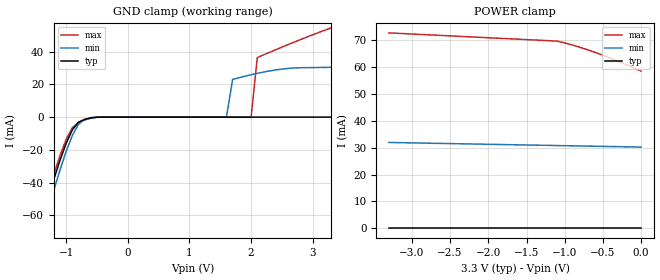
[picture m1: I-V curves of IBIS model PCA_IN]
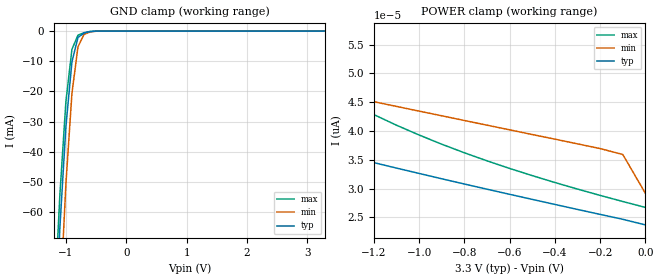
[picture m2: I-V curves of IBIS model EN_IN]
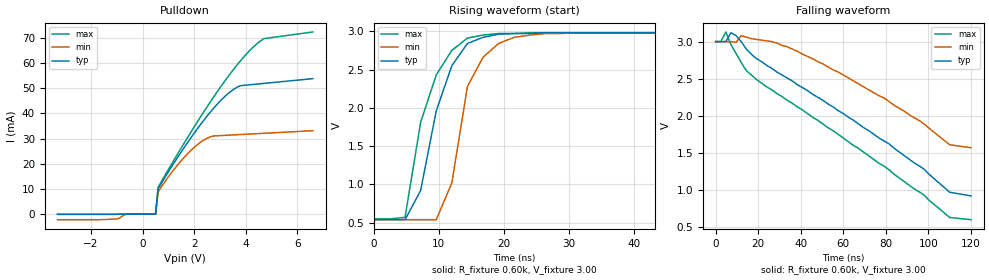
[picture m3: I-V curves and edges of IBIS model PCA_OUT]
| Philips Semiconductors Inc.
| Specialty Logic Group
| IBIS model of PCA9518
| Expandable 5-channel I2C Hub
[IBIS ver]   3.2
[File name]   pca9518.ibs
[File Rev]   1.0
[Date]   July 16, 2002
[Source]   Philips Semiconductors, Albuquerque
[Notes]   Generated by GMJ
PCA9518 IBIS MODEL
Because the PCA9518 is a repeater, not a buffer, this IBIS model does not model
the functionality of part correctly.  It only models unidirectional output
characteristics of the part. This is due to the fact that the input voltage
characteristics are affected by the voltage on the output side.
And as seen in the graph is a time dependent behavior.  This is illustrated
in the image Difference.png
[Disclaimer]
   (C) Copyright 2002 Philips Semiconductors
   All rights reserved
   Philips Semiconductors warrants and represents that the IBIS model
   identified herein is owned by Philips Semiconductors (PHILIPS). The
   model provided is not warranted as fully representing all of the
   operating characteristics and specifications of the semiconductor
   products to which the model relates.  Moreover, unless there is a
   signed, written agreement to the contrary, this IBIS model is
   furnished on an "as is" basis without support or warranty of any
   kind, either expressed or implied, regarding the use thereof, and
   PHILIPS specifically disclaims all implied warranties of
   merchantability and fitness of the model for any purpose.
   PHILIPS does not assume any liability arising out of the application
   or use of this IBIS model including infringement of patents and
   copyrights, nor does PHILIPS convey any license under its patents and
   copyrights or the rights of others.
   PHILIPS provides IBIS models as a service to our customers. You and
   your company shall not distribute, convey, sell, or give these models
   to anyone else without receiving prior written permission from
   PHILIPS.
   PHILIPS reserves the right to make changes without notice to these
   IBIS models to improve reliability, function, or design.
   Please be aware that your receipt and subsequent use of the IBIS
   information provided shall serve as acceptance of the terms and
   conditions of this agreement.  If you do not accept these terms,
   you should return or destroy the IBIS models and any other
   accompanying information immediately.
|   Component PCA9518
[Component]   PCA9518D
[Manufacturer]   Philips Semiconductors
[Package]
|[Package]   SO20
|   typ   min   max
R_pkg   5.95E-02   5.36E-02   6.59E-02
L_pkg   4.21E-09   3.07E-09   5.91E-09
C_pkg   0.910E-12  0.758E-12  1.110E-12
| Note:  All clock & data paths bidirectional.  IN/OUT choices arbitrary.
[Pin]  signal_name   model_name   R_pin   L_pin   C_pin
1   EXPSCL1   PCA_IN   5.75E-02  5.91E-09  1.050E-12
2   EXPSCL2   PCA_OUT   6.25E-02  4.85E-09  1.040E-12
3   SCL0   PCA_IN   6.59E-02  3.92E-09  0.861E-12
4   SDA0   PCA_IN   5.79E-02  3.32E-09  0.803E-12
5   SCL1   PCA_OUT   5.36E-02  3.07E-09  0.758E-12
6   SDA1   PCA_OUT   5.36E-02  3.07E-09  0.758E-12
7   EN1   EN_IN   5.79E-02  3.32E-09  0.803E-12
8   SCL2   POWER   6.59E-02  3.92E-09  0.861E-12
9   SDA2   PCA_OUT   6.25E-02  4.85E-09  1.040E-12
10   GND   PCA_OUT   5.75E-02  5.91E-09  1.110E-12
11   EN2   EN_IN   5.75E-02  5.91E-09  1.110E-12
12   SCL3   PCA_OUT   6.25E-02  4.85E-09  1.040E-12
13   SDA3   PCA_OUT   6.59E-02  3.92E-09  0.861E-12
14   EN3   EN_IN   5.79E-02  3.32E-09  0.803E-12
15   SCL4   PCA_OUT   5.36E-02  3.07E-09  0.758E-12
16   SDA4   PCA_OUT   5.36E-02  3.07E-09  0.758E-12
17   EN4   EN_IN   5.79E-02  3.32E-09  0.803E-12
18   EXPSDA1   PCA_IN   6.59E-02  3.92E-09  0.861E-12
19   EXPSDA2   PCA_OUT   6.25E-02  4.85E-09  1.040E-12
20   VCC   POWER   5.75E-02  5.91E-09  1.110E-12
[Component]   PCA9518PW
[Manufacturer]   Philips Semiconductors
[Package]
|[Package]   TSSOP20
|   typ   min   max
R_pkg   7.24E-02   6.63E-02   8.34E-02
L_pkg   2.47E-09   2.09E-09   3.18E-09
C_pkg   0.341E-12  0.282E-12  0.420E-12
| Note:  All clock & data paths bidirectional.  IN/OUT choices arbitrary.
[Pin]  signal_name   model_name   R_pin   L_pin   C_pin
1   EXPSCL1   PCA_IN   6.63E-02  3.18E-09  0.408E-12
2   EXPSCL2   PCA_OUT   6.67E-02  2.55E-09  0.398E-12
3   SCL0   PCA_IN   8.34E-02  2.35E-09  0.317E-12
4   SDA0   PCA_IN   7.44E-02  2.16E-09  0.293E-12
5   SCL1   PCA_OUT   7.10E-02  2.09E-09  0.282E-12
6   SDA1   PCA_OUT   7.10E-02  2.09E-09  0.282E-12
7   EN1   EN_IN   7.44E-02  2.16E-09  0.293E-12
8   SCL2   POWER   8.34E-02  2.35E-09  0.317E-12
9   SDA2   PCA_OUT   6.67E-02  2.55E-09  0.397E-12
10   GND   PCA_OUT   6.63E-02  3.18E-09  0.420E-12
11   EN2   EN_IN   6.63E-02  3.17E-09  0.420E-12
12   SCL3   PCA_OUT   6.67E-02  2.55E-09  0.397E-12
13   SDA3   PCA_OUT   8.34E-02  2.35E-09  0.317E-12
14   EN3   EN_IN   7.44E-02  2.16E-09  0.293E-12
15   SCL4   PCA_OUT   7.10E-02  2.09E-09  0.282E-12
16   SDA4   PCA_OUT   7.10E-02  2.09E-09  0.282E-12
17   EN4   EN_IN   7.44E-02  2.16E-09  0.293E-12
18   EXPSDA1   PCA_IN   8.34E-02  2.35E-09  0.317E-12
19   EXPSDA2   PCA_OUT   6.67E-02  2.55E-09  0.398E-12
20   VCC   POWER   6.63E-02  3.17E-09  0.420E-12
| Models and submodels in the file (3): PCA_IN (Input), EN_IN (Input), PCA_OUT (Open_drain)
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|   Model PCA_IN
[Model]   PCA_IN
Model_type   Input
Vinl =   0.50V
Vinh =   2.50V
C_comp   5.00pF   5.00pF   5.00pF
[Temperature Range]   27.00   70.00   0.000
[Voltage Range]   3.30V   3.00V   3.60V
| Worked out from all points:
|   GND clamp passes 1 mA (typ) near -0.66 V on its own axis
[GND_clamp]
| voltage   I(typ)   I(min)   I(max)
-3.3V     -340mA     -350mA     -330mA
-1.5V     -76.49mA   -84.37mA   -73.19mA
-1.4V     -63.24mA   -70.75mA   -59.96mA
-1V       -15.96mA   -20.9mA    -13.54mA
-900mV    -7.75mA    -11.17mA   -6.43mA
-800mV    -3.12mA    -4.33mA    -3.2mA
-700mV    -1.41mA    -1.29mA    -1.74mA
1.6V      29.23pA    32.44pA    29.06pA
1.7V      31.36pA    22.97mA    31.34pA
2V        37.97pA    25.86mA    38.69pA
2.1V      40.25pA    26.71mA    36.33mA
3.3V      73.63pA    30.39mA    54.51mA
[POWER_clamp]
| voltage   I(typ)   I(min)   I(max)
-3.3V     560pA      31.96mA    72.81mA
-1.1V     130pA      30.8mA     69.76mA
-1V       120pA      30.75mA    69.07mA
-900mV    110pA      30.7mA     68.29mA
-700mV    100pA      30.59mA    66.51mA
-600mV    98.17pA    30.54mA    65.52mA
-500mV    93.48pA    30.49mA    64.47mA
-300mV    84.89pA    30.39mA    62.22mA
0V        73.63pA    30.23mA    58.52mA
|   Model EN_IN
[Model]   EN_IN
Model_type   Input
Enable   Active-High
Vinl =   0.50V
Vinh =   2.50V
C_comp   5.00pF   5.00pF   5.00pF
[Temperature Range]   27.00   70.00   0.000
[Voltage Range]   3.30V   3.00V   3.60V
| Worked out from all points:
|   GND clamp passes 1 mA (typ) near -0.72 V on its own axis
[GND_clamp]
| voltage   I(typ)   I(min)   I(max)
-3.3V     -1.4A      -1.5A      -1.38A
-1.2V     -110mA     -140mA     -94.8mA
-1.1V     -65.23mA   -91.55mA   -54.4mA
-1V       -31.67mA   -50.72mA   -23.4mA
-900mV    -10.21mA   -20.66mA   -6.06mA
-800mV    -2.12mA    -5.24mA    -1.35mA
-700mV    -650uA     -1.09mA    -540uA
-600mV    -170uA     -300uA     -120uA
-500mV    -19.26uA   -44.66uA   -17.4uA
3.3V      23.67pA    37.76pA    -3.93nA
[POWER_clamp]
| voltage   I(typ)   I(min)   I(max)
-3.3V     62.39pA    62.57pA    200pA
-3V       56.74pA    60.02pA    150pA
-2.6V     50.46pA    56.65pA    100pA
-2.2V     45.18pA    53.32pA    75.29pA
-1.8V     40.59pA    50.01pA    58.19pA
-1.7V     39.52pA    49.18pA    54.97pA
-1.5V     37.45pA    47.54pA    49.44pA
-1.3V     35.47pA    45.91pA    44.86pA
-1V       32.62pA    43.45pA    39.3pA
-600mV    28.99pA    40.2pA     33.49pA
-100mV    24.65pA    35.91pA    27.74pA
0V        23.67pA    29.15pA    26.71pA
|   Model PCA_OUT
[Model]   PCA_OUT
Model_type   Open_drain
Polarity   Non-Inverting
C_comp   5.00pF   5.00pF   5.00pF
[Temperature Range]   27.00   70.00   0.000
[Voltage Range]   3.30V   3.00V   3.60V
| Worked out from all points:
|   rising waveform, R_fixture 0.60k, V_fixture 3.00: 20-80 % time 4.34ns typ, 3.77ns min, 4.43ns max; typ from 0.54 V to 2.99 V
|   falling waveform, R_fixture 0.60k, V_fixture 3.00: 20-80 % time 65.9ns typ, 50.1ns min, 72.2ns max; typ from 3 V to 0.92 V
[Pulldown]
| voltage   I(typ)   I(min)   I(max)
-3.3V     -100uA     -2.2mA     -1uA
-1V       -100uA     -1.9mA     -1uA
-600mV    -3.7uA     -67.5uA    -1uA
500mV     100pA      0A         0A
600mV     10.09mA    8.87mA     10.65mA
1.6V      26.33mA    22.43mA    28.07mA
2.1V      33.64mA    27.43mA    36.33mA
2.5V      39mA       30.18mA    42.69mA
3.3V      47.79mA    31.37mA    54.51mA
3.8V      51.06mA    31.64mA    61.02mA
4.7V      51.95mA    32.13mA    69.76mA
6.6V      53.85mA    33.16mA    72.39mA
[Ramp]
| variable   typ   min   max
dV/dt_r   1.65/3.64n   1.35/1.92n   1.95/4.04n
dV/dt_f   1.30/68.47n   0.96/53.14n   1.52/77.32n
R_load = 0.60k
[Rising Waveform]
R_fixture = 0.60k
V_fixture = 3.00
| time   V(typ)   V(min)   V(max)
0s        540mV      540mV      550mV
4.8ns     540mV      540mV      570mV
7.2ns     920mV      540mV      1.81V
9.6ns     1.96V      540mV      2.43V
12ns      2.55V      1.02V      2.75V
14.4ns    2.84V      2.28V      2.91V
16.8ns    2.92V      2.66V      2.95V
19.2ns    2.96V      2.84V      2.97V
26.4ns    2.98V      2.97V      2.98V
120ns     2.99V      2.99V      2.99V
[Falling Waveform]
R_fixture = 0.60k
V_fixture = 3.00
| time   V(typ)   V(min)   V(max)
0s        3V         3V         3V
2.4ns     3V         3V         3V
4.8ns     3V         3V         3.13V
7.2ns     3.12V      3V         2.96V
14.4ns    2.9V       3.06V      2.61V
33.6ns    2.51V      2.93V      2.21V
79.2ns    1.66V      2.24V      1.32V
98.4ns    1.27V      1.88V      920mV
110ns     970mV      1.61V      630mV
120ns     920mV      1.57V      600mV
